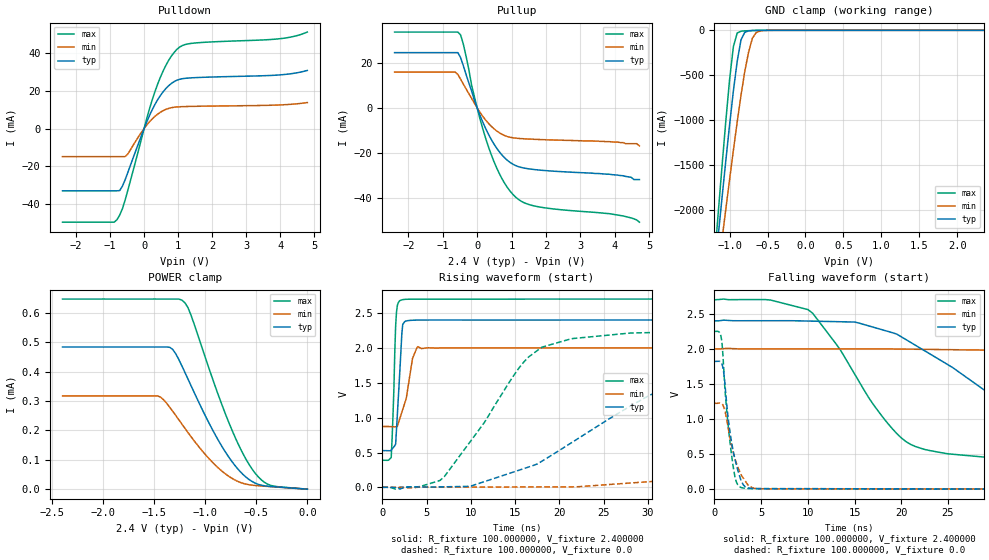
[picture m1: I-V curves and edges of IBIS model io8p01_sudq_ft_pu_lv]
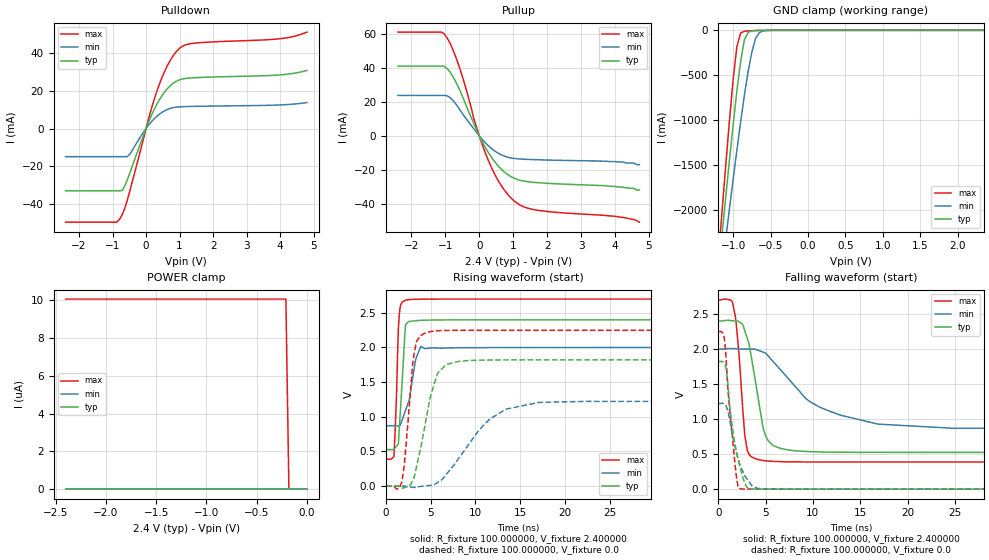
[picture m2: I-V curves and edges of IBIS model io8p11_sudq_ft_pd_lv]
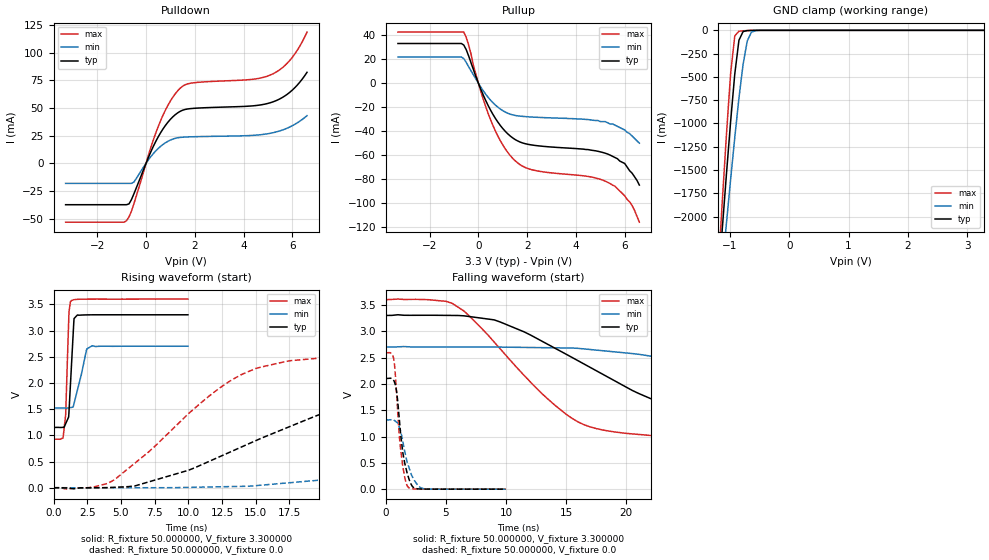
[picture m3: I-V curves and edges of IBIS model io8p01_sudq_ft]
|   stm32f0_440_wlcsp36 IBIS Model
[IBIS ver]   4.2
[File name]  stm32f0_440_wlcsp36.ibs
[File Rev]   1.0
[Date]   15-5-2013
[Source] Data Created at STMicroelectronics
[Notes]   File originated from ELDO simulations.
[Disclaimer]  This information is for modeling purpose only and is
   not guaranted. The information is subject to change without
   notice.
[Copyright] Copyright 2015 STMicroelectronics Inc.
[Component] stm32f0_440_wlcsp36
[Manufacturer] STMicroelectronics
[Package]
| variable   typ   min   max
R_pkg   0.0   NA   NA
L_pkg   0.0H   NA   NA
C_pkg   0.0F   NA   NA
[Pin] signal_name  model_name   R_pin   L_pin   C_pin
A6   PC13  io8p_sudq_tc
B6   PC14  io8p_sudq_tc
C6   PC15  io8p_sudq_tc
B5   PF0   io8p_sudq_ft
C5   PF1   io8p_sudq_ft
D5   NRST  ioreset_tc_v33
E5   VDDA  POWER
F6   PA0   io8p_sudq_ft
D4   PA1   io8p_sudq_ft
E4   PA2   io8p_sudq_ft
F5   PA3   io8p_sudq_ft
C3   PA4   io8p_sudq_ft
D3   PA5   io8p_sudq_ft
E3   PA6   io8p_sudq_ft
F4   PA7   io8p_sudq_ft
F3   PB0   io8p_sudq_ft
F2   PB1   io8p_sudq_ft
D2   PB2   io8p_sudq_ft
F1   VSS   GND
E1   VDD   POWER
E2   PA8   io8p_sudq_ft
D1   PA9   io8p_sudq_ft
C1   PA10  io8p_sudq_ft
C2   PA11  io8p_sudq_ft
A1   PA12  io8p_sudq_ft
B1   PA13  io8p_sudq_ft
B2   PA14  io8p_sudq_ft
A2   PA15  io8p_sudq_ft
B3   PB3   io8p_sudq_ft
A3   PB4   io8p_sudq_ft
E6   PB5   io8p_sudq_ft
C4   PB6   io8p_sudq_i2cin_lv_ft
A4   PB7   io8p_sudq_i2cin_lv_ft
B4   BOOT0 vpp_test_hv
D6   VSS   GND
A5   VDD   POWER
[Model Selector] io8p_sudq_ft
io8p01_sudq_ft_pd_lv  "SPEED01 2P0V, PD=40kOhm"
io8p01_sudq_ft_pu_lv  "SPEED01 2P0V, PU=40kOhm"
io8p01_sudq_ft_lv  "SPEED01 2P0V"
io8p10_sudq_ft_pd_lv  "SPEED10 2P0V, PD=40kOhm"
io8p10_sudq_ft_pu_lv  "SPEED10 2P0V, PU=40kOhm"
io8p10_sudq_ft_lv  "SPEED10 2P0V"
io8p11_sudq_ft_pd_lv  "SPEED11 2P0V, PD=40kOhm"
io8p11_sudq_ft_pu_lv  "SPEED11 2P0V, PU=40kOhm"
io8p11_sudq_ft_lv  "SPEED11 2P0V"
io8p01_sudq_ft_pd  "SPEED01, PD=40kOhm"
io8p01_sudq_ft_pu  "SPEED01, PU=40kOhm"
io8p01_sudq_ft  "SPEED01"
io8p10_sudq_ft_pd  "SPEED10, PD=40kOhm"
io8p10_sudq_ft_pu  "SPEED10, PU=40kOhm"
io8p10_sudq_ft  "SPEED10"
io8p11_sudq_ft_pd  "SPEED11, PD=40kOhm"
io8p11_sudq_ft_pu  "SPEED11, PU=40kOhm"
io8p11_sudq_ft  "SPEED11"
[Model Selector] io8p_sudq_i2cin_lv_ft
io8p01_sudq_i2cin_lv_ft_pd_lv  "SPEED01 2P0V, PD=40kOhm"
io8p01_sudq_i2cin_lv_ft_pu_lv  "SPEED01 2P0V, PU=40kOhm"
io8p01_sudq_i2cin_lv_ft_lv  "SPEED01 2P0V"
io8p10_sudq_i2cin_lv_ft_pd_lv  "SPEED10 2P0V, PD=40kOhm"
io8p10_sudq_i2cin_lv_ft_pu_lv  "SPEED10 2P0V, PU=40kOhm"
io8p10_sudq_i2cin_lv_ft_lv  "SPEED10 2P0V"
io8p11_sudq_i2cin_lv_ft_pd_lv  "SPEED11 2P0V, PD=40kOhm"
io8p11_sudq_i2cin_lv_ft_pu_lv  "SPEED11 2P0V, PU=40kOhm"
io8p11_sudq_i2cin_lv_ft_lv  "SPEED11 2P0V"
io8p01_sudq_i2cin_lv_ft_pd  "SPEED01, PD=40kOhm"
io8p01_sudq_i2cin_lv_ft_pu  "SPEED01, PU=40kOhm"
io8p01_sudq_i2cin_lv_ft  "SPEED01"
io8p10_sudq_i2cin_lv_ft_pd  "SPEED10, PD=40kOhm"
io8p10_sudq_i2cin_lv_ft_pu  "SPEED10, PU=40kOhm"
io8p10_sudq_i2cin_lv_ft  "SPEED10"
io8p11_sudq_i2cin_lv_ft_pd  "SPEED11, PD=40kOhm"
io8p11_sudq_i2cin_lv_ft_pu  "SPEED11, PU=40kOhm"
io8p11_sudq_i2cin_lv_ft  "SPEED11"
[Model Selector] io8p_sudq_tc
io8p01_sudq_tc_pd_lv  "SPEED01 2P0V, PD=40kOhm"
io8p01_sudq_tc_pu_lv  "SPEED01 2P0V, PU=40kOhm"
io8p01_sudq_tc_lv  "SPEED01 2P0V"
io8p10_sudq_tc_pd_lv  "SPEED10 2P0V, PD=40kOhm"
io8p10_sudq_tc_pu_lv  "SPEED10 2P0V, PU=40kOhm"
io8p10_sudq_tc_lv  "SPEED10 2P0V"
io8p11_sudq_tc_pd_lv  "SPEED11 2P0V, PD=40kOhm"
io8p11_sudq_tc_pu_lv  "SPEED11 2P0V, PU=40kOhm"
io8p11_sudq_tc_lv  "SPEED11 2P0V"
io8p01_sudq_tc_pd  "SPEED01, PD=40kOhm"
io8p01_sudq_tc_pu  "SPEED01, PU=40kOhm"
io8p01_sudq_tc  "SPEED01"
io8p10_sudq_tc_pd  "SPEED10, PD=40kOhm"
io8p10_sudq_tc_pu  "SPEED10, PU=40kOhm"
io8p10_sudq_tc  "SPEED10"
io8p11_sudq_tc_pd  "SPEED11, PD=40kOhm"
io8p11_sudq_tc_pu  "SPEED11, PU=40kOhm"
io8p11_sudq_tc  "SPEED11"
[Model Selector] ioreset_tc_v33
ioreset_tc_v33_pu_lv  "IORESET 2V + PU=40kOhm"
ioreset_tc_v33_nopu_lv  "IORESET 2V"
ioreset_tc_v33_pu  "IORESET + PU=40kOhm"
ioreset_tc_v33_nopu  "IORESET"
[Model Selector] vpp_test_hv
vpp_test_hv_3p3  "Input Buffer"
vpp_test_hv_2p4  "Input Buffer 2P0V"
| Models and submodels in the file (60): io8p01_sudq_ft_pd_lv (I/O), io8p01_sudq_ft_pu_lv (I/O), io8p01_sudq_ft_lv (I/O), io8p10_sudq_ft_pd_lv (I/O), io8p10_sudq_ft_pu_lv (I/O), io8p10_sudq_ft_lv (I/O), io8p11_sudq_ft_pd_lv (I/O), io8p11_sudq_ft_pu_lv (I/O), io8p11_sudq_ft_lv (I/O), io8p01_sudq_ft_pd (I/O), io8p01_sudq_ft_pu (I/O), io8p01_sudq_ft (I/O), io8p10_sudq_ft_pd (I/O), io8p10_sudq_ft_pu (I/O), io8p10_sudq_ft (I/O), io8p11_sudq_ft_pd (I/O), io8p11_sudq_ft_pu (I/O), io8p11_sudq_ft (I/O), io8p01_sudq_i2cin_lv_ft_pd_lv (I/O), io8p01_sudq_i2cin_lv_ft_pu_lv (I/O), io8p01_sudq_i2cin_lv_ft_lv (I/O), io8p10_sudq_i2cin_lv_ft_pd_lv (I/O), io8p10_sudq_i2cin_lv_ft_pu_lv (I/O), io8p10_sudq_i2cin_lv_ft_lv (I/O), io8p11_sudq_i2cin_lv_ft_pd_lv (I/O), io8p11_sudq_i2cin_lv_ft_pu_lv (I/O), io8p11_sudq_i2cin_lv_ft_lv (I/O), io8p01_sudq_i2cin_lv_ft_pd (I/O), io8p01_sudq_i2cin_lv_ft_pu (I/O), io8p01_sudq_i2cin_lv_ft (I/O), io8p10_sudq_i2cin_lv_ft_pd (I/O), io8p10_sudq_i2cin_lv_ft_pu (I/O), io8p10_sudq_i2cin_lv_ft (I/O), io8p11_sudq_i2cin_lv_ft_pd (I/O), io8p11_sudq_i2cin_lv_ft_pu (I/O), io8p11_sudq_i2cin_lv_ft (I/O), io8p01_sudq_tc_pd_lv (I/O), io8p01_sudq_tc_pu_lv (I/O), io8p01_sudq_tc_lv (I/O), io8p10_sudq_tc_pd_lv (I/O), io8p10_sudq_tc_pu_lv (I/O), io8p10_sudq_tc_lv (I/O), io8p11_sudq_tc_pd_lv (I/O), io8p11_sudq_tc_pu_lv (I/O), io8p11_sudq_tc_lv (I/O), io8p01_sudq_tc_pd (I/O), io8p01_sudq_tc_pu (I/O), io8p01_sudq_tc (I/O), io8p10_sudq_tc_pd (I/O), io8p10_sudq_tc_pu (I/O), io8p10_sudq_tc (I/O), io8p11_sudq_tc_pd (I/O), io8p11_sudq_tc_pu (I/O), io8p11_sudq_tc (I/O), ioreset_tc_v33_pu_lv (I/O_open_drain), ioreset_tc_v33_nopu_lv (I/O_open_drain), ioreset_tc_v33_pu (I/O_open_drain), ioreset_tc_v33_nopu (I/O_open_drain), vpp_test_hv_2p4 (Input), vpp_test_hv_3p3 (Input)
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|   Model io8p01_sudq_ft_pu_lv
[Model]  io8p01_sudq_ft_pu_lv
Model_type I/O
Polarity   Non-Inverting
Enable   Active-Low
Vinl =   0.720000V
Vinh =   1.680000V
Vmeas =  1.200000V
Cref =   50.000000pF
Rref =   100.000000M
Vref =   0.0V
C_comp   1.970100pF   1.887900pF   2.069400pF
[Temperature Range]   25.000000   0.125000k   -40.000000
[Pullup Reference]   2.400000V   2.000000V   2.700000V
[Pulldown Reference]   0.0V   0.0V   0.0V
[POWER Clamp Reference]   2.400000V   2.000000V   2.700000V
[GND Clamp Reference]   0.0V   0.0V   0.0V
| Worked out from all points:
|   slope of the pulldown table from 0 to 0.36 V, typ, clamps not added: 25.5 ohm
|   slope of the pullup table from 0 to 0.36 V, typ, clamps not added: 28.4 ohm
|   GND clamp passes 1 mA (typ) near -0.64 V on its own axis
|   rising waveform, R_fixture 100.000000, V_fixture 2.400000: 20-80 % time 497ps typ, 1.06ns min, 335ps max; typ from 0.527 V to 2.4 V
|   rising waveform, R_fixture 100.000000, V_fixture 0.0: 20-80 % time 14.6ns typ, 42.8ns min, 7.27ns max; typ from 0.001 V to 1.82 V
|   falling waveform, R_fixture 100.000000, V_fixture 2.400000: 20-80 % time 12.9ns typ, 32.5ns min, 7.06ns max; typ from 2.4 V to 0.527 V
|   falling waveform, R_fixture 100.000000, V_fixture 0.0: 20-80 % time 1.16ns typ, 1.4ns min, 913ps max; typ from 1.82 V to 0.001 V
[Pulldown]
|Voltage   I(typ)   I(min)   I(max)
-2.4V     -33.16mA   -14.98mA   -49.86mA
-880mV    -33.16mA   -14.98mA   -49.86mA
-800mV    -33.16mA   -14.98mA   -48.55mA
-640mV    -30.75mA   -14.98mA   -42.77mA
-480mV    -23.43mA   -13.57mA   -32.92mA
80mV      3.651mA    1.905mA    5.506mA
400mV     15.37mA    7.665mA    23.73mA
720mV     22.75mA    10.69mA    36.23mA
1.04V     26.18mA    11.57mA    43.27mA
1.52V     27.09mA    11.81mA    45.55mA
4V        28.55mA    12.55mA    47.81mA
4.8V      30.9mA     13.81mA    51.31mA
[Pullup]
|Voltage   I(typ)   I(min)   I(max)
-2.4V     24.57mA    15.91mA    33.73mA
-640mV    24.57mA    15.91mA    33.73mA
-480mV    22.32mA    12.71mA    32.43mA
-400mV    18.71mA    10.52mA    28.28mA
-160mV    7.421mA    4.162mA    10.02mA
0V        81fA       15.2pA     0A
320mV     -11.51mA   -6.781mA   -16.98mA
720mV     -21mA      -11.8mA    -31.53mA
1.2V      -26.24mA   -13.65mA   -40.83mA
1.76V     -27.69mA   -14.12mA   -44.07mA
3.84V     -29.6mA    -15.1mA    -47.2mA
4.72V     -32mA      -17mA      -51mA
[GND_clamp]
|Voltage   I(typ)   I(min)   I(max)
-2.4V     -9.788A    -9.782A    -9.734A
-1.2V     -2.718A    -3.02A     -2.568A
-1.15V    -2.29A     -2.675A    -2.036A
-1.1V     -1.868A    -2.333A    -1.515A
-1.05V    -1.454A    -1.995A    -1.012A
-950mV    -674.5mA   -1.337A    -180.5mA
-900mV    -345.2mA   -1.023A    -29.72mA
-850mV    -106.4mA   -726mA     -10.13mA
-750mV    -6.396mA   -244mA     -4.026mA
-700mV    -2.558mA   -88.61mA   -2.329mA
-600mV    -416uA     -7.739mA   -368uA
2.35V     0A         0A         0A
[POWER_clamp]
|Voltage   I(typ)   I(min)   I(max)
-2.4V     483.8uA    317.4uA    647uA
-1.47V    483.8uA    317.4uA    647uA
-1.32V    475.6uA    265.2uA    647uA
-1.23V    419.7uA    221.6uA    643.3uA
-1.17V    374.8uA    192.7uA    617.6uA
-1.14V    352.1uA    178.7uA    591.9uA
-840mV    147uA      62.15uA    289.6uA
-690mV    72.24uA    27.76uA    162.7uA
-540mV    25.74uA    13.55uA    67.63uA
-450mV    13.38uA    10.75uA    31.36uA
-360mV    9.231uA    8.535uA    12.97uA
0V        0A         0A         0A
[Ramp]
| variable   typ   min   max
dV/dt_r  1.09269/14.55881n   0.73353/42.71845n   1.34908/7.26325n
dV/dt_f  1.12400/12.83842n   0.67649/32.44923n   1.38689/7.04961n
R_load = 100.000000
[Rising Waveform]
R_fixture= 100.000000
V_fixture= 2.400000
V_fixture_min= 2.000000
V_fixture_max= 2.700000
|time   V(typ)   V(min)   V(max)
0s        526.5mV    872.5mV    388.6mV
1.001ns   534.8mV    870.7mV    429.3mV
1.301ns   581.8mV    869.1mV    1.401V
1.502ns   620.7mV    868.5mV    2.316V
1.602ns   841mV      868.2mV    2.522V
2.102ns   1.968V     1.038V     2.685V
2.302ns   2.337V     1.118V     2.692V
3.403ns   2.396V     1.846V     2.698V
4.004ns   2.398V     2.018V     2.698V
49.85ns   2.4V       2V         2.7V
[Rising Waveform]
R_fixture= 100.000000
V_fixture= 0.0
V_fixture_min= 0.0
V_fixture_max= 0.0
|time   V(typ)   V(min)   V(max)
0s        1.057mV    1.357mV    941.6uV
6.507ns   6.739mV    4.851mV    98.8mV
15.52ns   249.4mV    5.766mV    1.725V
18.02ns   374.6mV    6.657mV    2.009V
28.03ns   1.166V     62.6mV     2.213V
34.53ns   1.553V     120.9mV    2.23V
43.04ns   1.725V     229mV      2.248V
79.08ns   1.822V     883.8mV    2.25V
103.1ns   1.822V     1.116V     2.249V
249.2ns   1.822V     1.224V     2.25V
[Falling Waveform]
R_fixture= 100.000000
V_fixture= 2.400000
V_fixture_min= 2.000000
V_fixture_max= 2.700000
|time   V(typ)   V(min)   V(max)
0s        2.4V       2V         2.7V
10.01ns   2.397V     2V         2.56V
15.02ns   2.383V     2V         1.64V
20.02ns   2.171V     1.997V     729.2mV
29.53ns   1.353V     1.982V     451.1mV
38.04ns   762.8mV    1.926V     413.2mV
57.06ns   576.4mV    1.555V     391.8mV
84.58ns   537.8mV    1.049V     388.5mV
102.6ns   530.3mV    958.5mV    388.5mV
249.2ns   526.5mV    872.5mV    388.6mV
[Falling Waveform]
R_fixture= 100.000000
V_fixture= 0.0
V_fixture_min= 0.0
V_fixture_max= 0.0
|time   V(typ)   V(min)   V(max)
0s        1.822V     1.224V     2.25V
700.7ps   1.803V     1.224V     2.18V
800.8ps   1.785V     1.217V     2.098V
1.001ns   1.655V     1.167V     1.705V
1.401ns   1.091V     924.7mV    994.1mV
1.802ns   692.7mV    650.1mV    517.8mV
2.302ns   370.4mV    389.6mV    121.1mV
2.903ns   110.3mV    193.7mV    21.86mV
4.605ns   7.762mV    8.133mV    8.175mV
49.85ns   1.057mV    1.357mV    941.6uV
|   Model io8p11_sudq_ft_pd_lv
[Model]  io8p11_sudq_ft_pd_lv
Model_type I/O
Polarity   Non-Inverting
Enable   Active-Low
Vinl =   0.720000V
Vinh =   1.680000V
Vmeas =  1.200000V
Cref =   50.000000pF
Rref =   100.000000M
Vref =   0.0V
C_comp   1.970100pF   1.887900pF   2.069400pF
[Temperature Range]   25.000000   0.125000k   -40.000000
[Pullup Reference]   2.400000V   2.000000V   2.700000V
[Pulldown Reference]   0.0V   0.0V   0.0V
[POWER Clamp Reference]   2.400000V   2.000000V   2.700000V
[GND Clamp Reference]   0.0V   0.0V   0.0V
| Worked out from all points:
|   slope of the pulldown table from 0 to 0.36 V, typ, clamps not added: 25.5 ohm
|   slope of the pullup table from 0 to 0.36 V, typ, clamps not added: 28.4 ohm
|   GND clamp passes 1 mA (typ) near -0.64 V on its own axis
|   rising waveform, R_fixture 100.000000, V_fixture 2.400000: 20-80 % time 509ps typ, 1.05ns min, 339ps max; typ from 0.525 V to 2.4 V
|   rising waveform, R_fixture 100.000000, V_fixture 0.0: 20-80 % time 1.79ns typ, 4.5ns min, 864ps max; typ from 0 V to 1.82 V
|   falling waveform, R_fixture 100.000000, V_fixture 2.400000: 20-80 % time 1.38ns typ, 6ns min, 772ps max; typ from 2.4 V to 0.525 V
|   falling waveform, R_fixture 100.000000, V_fixture 0.0: 20-80 % time 1.16ns typ, 1.4ns min, 850ps max; typ from 1.82 V to 0 V
[Pulldown]
|Voltage   I(typ)   I(min)   I(max)
-2.4V     -33.16mA   -14.98mA   -49.86mA
-880mV    -33.16mA   -14.98mA   -49.86mA
-800mV    -33.16mA   -14.98mA   -48.55mA
-640mV    -30.75mA   -14.98mA   -42.76mA
-480mV    -23.43mA   -13.57mA   -32.92mA
80mV      3.651mA    1.905mA    5.506mA
400mV     15.37mA    7.665mA    23.73mA
720mV     22.75mA    10.69mA    36.23mA
1.04V     26.18mA    11.57mA    43.27mA
1.52V     27.09mA    11.81mA    45.55mA
4V        28.55mA    12.55mA    47.81mA
4.8V      30.9mA     13.81mA    51.31mA
[Pullup]
|Voltage   I(typ)   I(min)   I(max)
-2.4V     41.23mA    23.94mA    61.35mA
-1.12V    41.23mA    23.94mA    61.35mA
-960mV    40.07mA    23.8mA     58.26mA
-800mV    35.79mA    21.42mA    51.95mA
-560mV    26.31mA    15.01mA    38.92mA
-160mV    7.338mA    4.152mA    10.02mA
240mV     -8.977mA   -5.327mA   -13.21mA
640mV     -19.51mA   -11.09mA   -29.16mA
1.04V     -25.15mA   -13.38mA   -38.61mA
1.68V     -27.56mA   -14.07mA   -43.82mA
4V        -29.9mA    -15.2mA    -47.5mA
4.72V     -32mA      -17mA      -51mA
[GND_clamp]
|Voltage   I(typ)   I(min)   I(max)
-2.4V     -9.788A    -9.782A    -9.734A
-1.2V     -2.718A    -3.021A    -2.568A
-1.15V    -2.29A     -2.675A    -2.036A
-1.1V     -1.868A    -2.333A    -1.515A
-1.05V    -1.454A    -1.995A    -1.012A
-950mV    -674.5mA   -1.337A    -180.6mA
-900mV    -345.2mA   -1.023A    -29.74mA
-850mV    -106.4mA   -726mA     -10.14mA
-750mV    -6.411mA   -244mA     -4.042mA
-700mV    -2.572mA   -88.62mA   -2.346mA
-600mV    -429.6uA   -7.75mA    -383.5uA
2.35V     59.77uA    46.33uA    66.89uA
[POWER_clamp]
|Voltage   I(typ)   I(min)   I(max)
-2.4V     0A         0A         10.06uA
-210mV    0A         0A         10.06uA
-180mV    0A         0A         0A
0V        0A         0A         0A
[Ramp]
| variable   typ   min   max
dV/dt_r  1.09218/1.79238n   0.73266/4.49807n   1.34886/0.85997n
dV/dt_f  1.12444/1.38128n   0.67760/5.98085n   1.38699/0.77171n
R_load = 100.000000
[Rising Waveform]
R_fixture= 100.000000
V_fixture= 2.400000
V_fixture_min= 2.000000
V_fixture_max= 2.700000
|time   V(typ)   V(min)   V(max)
0s        524.8mV    868.7mV    387.2mV
900.9ps   532.4mV    867.1mV    423.6mV
1.201ns   575.3mV    865.9mV    1.359V
1.401ns   611.4mV    865.5mV    2.286V
1.602ns   1.042V     875.4mV    2.59V
2.202ns   2.327V     1.094V     2.683V
2.603ns   2.374V     1.24V      2.691V
3.303ns   2.385V     1.812V     2.695V
3.904ns   2.392V     2.015V     2.697V
49.85ns   2.399V     1.999V     2.699V
[Rising Waveform]
R_fixture= 100.000000
V_fixture= 0.0
V_fixture_min= 0.0
V_fixture_max= 0.0
|time   V(typ)   V(min)   V(max)
0s        -34.41uV   -16.09uV   -30.77uV
1.802ns   -29.45mV   -740.5uV   67.35mV
3.103ns   111mV      -21.8mV    1.872V
3.403ns   265.9mV    -17.88mV   2.083V
4.505ns   973.4mV    1.615mV    2.214V
5.706ns   1.601V     43.39mV    2.239V
6.707ns   1.75V      161.3mV    2.245V
10.71ns   1.817V     848.5mV    2.248V
13.51ns   1.82V      1.112V     2.248V
49.85ns   1.82V      1.221V     2.248V
[Falling Waveform]
R_fixture= 100.000000
V_fixture= 2.400000
V_fixture_min= 2.000000
V_fixture_max= 2.700000
|time   V(typ)   V(min)   V(max)
0s        2.399V     1.999V     2.699V
1.502ns   2.401V     2.006V     2.669V
1.902ns   2.399V     2.002V     2.364V
2.903ns   2.22V      1.998V     687.3mV
4.004ns   1.477V     1.993V     430.5mV
5.205ns   707.5mV    1.911V     401.7mV
7.508ns   556.9mV    1.561V     389.5mV
10.81ns   530.5mV    1.163V     387.2mV
16.82ns   524.9mV    928.9mV    387.2mV
49.85ns   524.8mV    868.7mV    387.2mV
[Falling Waveform]
R_fixture= 100.000000
V_fixture= 0.0
V_fixture_min= 0.0
V_fixture_max= 0.0
|time   V(typ)   V(min)   V(max)
0s        1.82V      1.221V     2.248V
700.7ps   1.782V     1.213V     2.099V
1.101ns   1.38V      1.068V     1.302V
1.301ns   1.08V      922.8mV    1.007V
1.802ns   621.8mV    592.1mV    322mV
2.102ns   428.2mV    431.4mV    33.52mV
2.302ns   319.1mV    346.1mV    4.266mV
3.103ns   16.96mV    133.5mV    1.213mV
4.605ns   776.8uV    5.445mV    417.8uV
49.85ns   -34.41uV   -16.09uV   -30.77uV
|   Model io8p01_sudq_ft
[Model]  io8p01_sudq_ft
Model_type I/O
Polarity   Non-Inverting
Enable   Active-Low
Vinl =   0.990000V
Vinh =   2.310000V
Vmeas =  1.650000V
Cref =   50.000000pF
Rref =   100.000000M
Vref =   0.0V
C_comp   1.970900pF   1.892300pF   2.063200pF
[Temperature Range]   25.000000   0.125000k   -40.000000
[Pullup Reference]   3.300000V   2.700000V   3.600000V
[Pulldown Reference]   0.0V   0.0V   0.0V
[POWER Clamp Reference]   3.300000V   2.700000V   3.600000V
[GND Clamp Reference]   0.0V   0.0V   0.0V
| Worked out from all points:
|   slope of the pulldown table from 0 to 0.495 V, typ, clamps not added: 20.9 ohm
|   slope of the pullup table from 0 to 0.495 V, typ, clamps not added: 22.2 ohm
|   GND clamp passes 1 mA (typ) near -0.64 V on its own axis
|   rising waveform, R_fixture 50.000000, V_fixture 3.300000: 20-80 % time 269ps typ, 640ps min, 200ps max; typ from 1.15 V to 3.3 V
|   rising waveform, R_fixture 50.000000, V_fixture 0.0: 20-80 % time 12.5ns typ, 30.4ns min, 7.06ns max; typ from 0 V to 2.1 V
|   falling waveform, R_fixture 50.000000, V_fixture 3.300000: 20-80 % time 10.9ns typ, 22.8ns min, 6.88ns max; typ from 3.3 V to 1.15 V
|   falling waveform, R_fixture 50.000000, V_fixture 0.0: 20-80 % time 666ps typ, 862ps min, 543ps max; typ from 2.1 V to 0 V
[Pulldown]
|Voltage   I(typ)   I(min)   I(max)
-3.3V     -37.45mA   -18.2mA    -53.24mA
-800mV    -37.45mA   -18.2mA    -51.9mA
-700mV    -36.7mA    -18.2mA    -48.48mA
-500mV    -27.71mA   -17.01mA   -36.66mA
200mV     10.57mA    6.084mA    14.57mA
500mV     23.91mA    13.38mA    33.24mA
900mV     37.17mA    19.88mA    52.48mA
1.3V      45.55mA    23.01mA    65.5mA
1.8V      49.29mA    23.83mA    72.18mA
5.1V      54.68mA    27.07mA    79.72mA
5.9V      64.2mA     32.82mA    93.01mA
6.6V      82.13mA    42.97mA    118.4mA
[Pullup]
|Voltage   I(typ)   I(min)   I(max)
-3.3V     33.18mA    21.9mA     42.7mA
-600mV    31.87mA    20.57mA    42.7mA
-400mV    22.78mA    13.76mA    31.89mA
100mV     -5.13mA    -3.299mA   -6.952mA
500mV     -22.5mA    -14.16mA   -30.52mA
900mV     -35.28mA   -21.55mA   -48mA
1.4V      -45.55mA   -26.41mA   -62.54mA
2.2V      -51.57mA   -28.22mA   -72.25mA
5.4V      -60mA      -34mA      -83.7mA
6V        -67mA      -39mA      -94mA
6.2V      -73mA      -42mA      -99mA
6.6V      -85mA      -50mA      -116mA
[GND_clamp]
|Voltage   I(typ)   I(min)   I(max)
-3.3V     -9.525A    -9.501A    -9.513A
-1.2V     -2.719A    -3.023A    -2.568A
-1.13V    -2.122A    -2.541A    -1.826A
-1.06V    -1.537A    -2.065A    -1.111A
-990mV    -975.7mA   -1.599A    -462mA
-920mV    -467.4mA   -1.149A    -59mA
-850mV    -106.6mA   -727.3mA   -10.11mA
-780mV    -13.06mA   -365.4mA   -5.254mA
-710mV    -3.045mA   -114.8mA   -2.635mA
-640mV    -943.2uA   -20.16mA   -905.7uA
-570mV    -199.4uA   -3.959mA   -156.8uA
3.28V     0A         0A         0A
[POWER_clamp]
|Voltage   I(typ)   I(min)   I(max)
-3.28V    0A         0A         0A
0V        0A         0A         0A
[Ramp]
| variable   typ   min   max
dV/dt_r  1.26240/12.53718n   0.78948/30.37625n   1.55460/7.05051n
dV/dt_f  1.28952/10.93890n   0.70650/22.81705n   1.60469/6.86180n
R_load = 50.000000
[Rising Waveform]
R_fixture= 50.000000
V_fixture= 3.300000
V_fixture_min= 2.700000
V_fixture_max= 3.600000
|time   V(typ)   V(min)   V(max)
0s        1.151V     1.522V     925.5mV
720.7ps   1.153V     1.522V     979.3mV
900.9ps   1.222V     1.52V      1.393V
1.141ns   1.422V     1.523V     3.312V
1.261ns   1.999V     1.529V     3.554V
1.522ns   3.228V     1.605V     3.588V
1.762ns   3.294V     1.851V     3.595V
2.462ns   3.298V     2.646V     3.599V
2.863ns   3.3V       2.708V     3.599V
9.97ns    3.3V       2.7V       3.6V
[Rising Waveform]
R_fixture= 50.000000
V_fixture= 0.0
V_fixture_min= 0.0
V_fixture_max= 0.0
|time   V(typ)   V(min)   V(max)
0s        2.028nV    11.57nV    2.55nV
4.505ns   8.246mV    23.61uV    149.8mV
10.01ns   333.3mV    6.624mV    1.413V
14.01ns   785.5mV    26.06mV    2.168V
22.52ns   1.625V     206.1mV    2.53V
28.03ns   1.898V     345.1mV    2.568V
39.54ns   2.061V     685.1mV    2.588V
55.56ns   2.101V     1.054V     2.592V
75.08ns   2.103V     1.24V      2.591V
249.2ns   2.104V     1.316V     2.591V
[Falling Waveform]
R_fixture= 50.000000
V_fixture= 3.300000
V_fixture_min= 2.700000
V_fixture_max= 3.600000
|time   V(typ)   V(min)   V(max)
0s        3.3V       2.7V       3.6V
5.506ns   3.3V       2.701V     3.532V
9.009ns   3.216V     2.7V       2.797V
13.01ns   2.808V     2.688V     1.811V
16.02ns   2.437V     2.675V     1.275V
22.52ns   1.673V     2.511V     1.015V
30.53ns   1.307V     2.227V     958.1mV
45.05ns   1.189V     1.779V     932.1mV
69.57ns   1.157V     1.587V     925.7mV
249.2ns   1.151V     1.522V     925.5mV
[Falling Waveform]
R_fixture= 50.000000
V_fixture= 0.0
V_fixture_min= 0.0
V_fixture_max= 0.0
|time   V(typ)   V(min)   V(max)
0s        2.104V     1.316V     2.591V
660.7ps   2.062V     1.315V     2.466V
900.9ps   1.84V      1.273V     1.796V
1.141ns   1.275V     1.165V     952.9mV
1.261ns   977.3mV    1.075V     694.5mV
1.602ns   464.8mV    685.7mV    192.5mV
1.862ns   238.4mV    452mV      36.35mV
2.282ns   34.71mV    203.8mV    5.722mV
3.103ns   2.027mV    11.23mV    1.089mV
9.97ns    2.028nV    11.57nV    2.55nV
